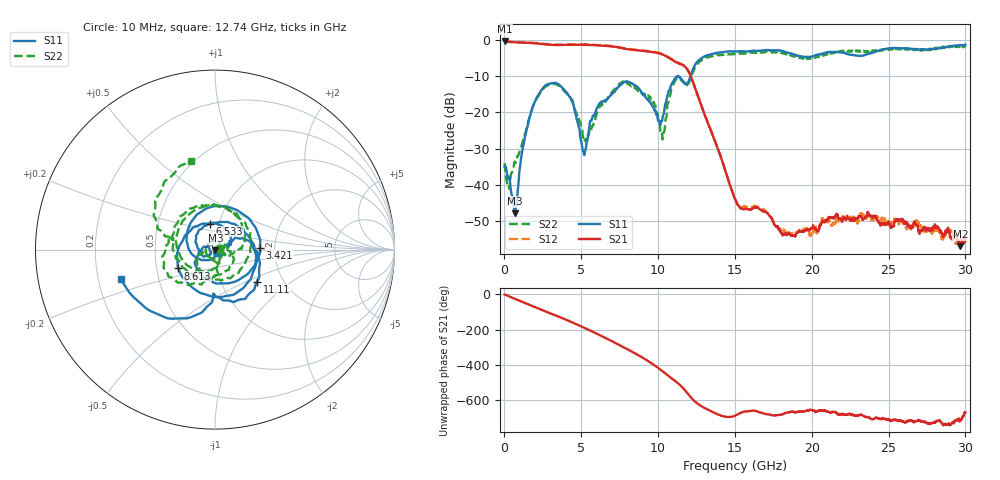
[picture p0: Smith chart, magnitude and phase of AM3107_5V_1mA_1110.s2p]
# Hz S DB R 50.0
!freq dBS11 angS11 dBS21 angS21 dBS12 angS12 dBS22 angS22
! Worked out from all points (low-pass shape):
!   1601 points, 10 MHz to 30 GHz, reference 50 ohm
!   highest |S21| = -0.16 dB at 10 MHz (marker M1); lowest = -57.1 dB at 29.68 GHz (marker M2)
!   |S21| within 3 dB of the highest: start of sweep to 9.478 GHz
!   lowest |S11| = -48.0 dB at 666 MHz (marker M3), VSWR 1.01, Z = 50.3 - j0.294 ohm
!   |S11| at or under -10 dB: start of sweep to 11.26 GHz; 11.33 GHz to 12.11 GHz (779.4 MHz wide, 6.65 % of centre)
!   |S22| runs from -41.2 to -1.5 dB; largest |S21 - S12| = 0.014
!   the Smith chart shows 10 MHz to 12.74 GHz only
!   S11 on the Smith chart (normalised r, x): 10 MHz: 1.02, -0.03; 3.421 GHz: 1.67, +0.03; 6.533 GHz: 0.91, +0.27; 8.613 GHz: 0.65, -0.14; 11.11 GHz: 1.48, -0.58; 12.74 GHz: 0.30, -0.14
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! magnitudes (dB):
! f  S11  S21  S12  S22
! 10 MHz  -35.1  -0.2  0.0  -34.1
! 253.7 MHz  -38.5  -0.4  -0.4  -40.2
! 666 MHz  -48.0  -0.6  -0.5  -33.6
! 1.809 GHz  -18.8  -0.8  -0.7  -18.8
! 3.421 GHz  -12.0  -1.3  -1.2  -12.3
! 4.377 GHz  -16.8  -1.3  -1.2  -16.6
! 5.015 GHz  -28.5  -1.3  -1.2  -24.0
! 5.352 GHz  -28.3  -1.3  -1.2  -27.9
! 6.533 GHz  -16.7  -1.5  -1.4  -16.8
! 7.695 GHz  -11.8  -2.2  -2.1  -11.4
! 8.613 GHz  -12.8  -2.8  -2.7  -13.7
! 10.02 GHz  -22.4  -3.6  -3.4  -22.2
! 10.32 GHz  -20.8  -4.0  -3.9  -26.6
! 11.11 GHz  -10.6  -5.9  -5.8  -11.1
! 11.87 GHz  -12.1  -7.9  -7.8  -12.4
! 12.74 GHz  -5.2  -17.2  -17.1  -5.8
! 15.01 GHz  -3.1  -44.0  -44.0  -3.8
! 18.14 GHz  -3.0  -54.0  -52.7  -3.6
! 20.01 GHz  -4.6  -52.2  -53.0  -5.0
! 25.01 GHz  -2.3  -50.4  -50.5  -2.6
! 29.68 GHz  -1.3  -57.1  -55.2  -1.7
! 30 GHz  -1.2  -55.4  -54.8  -1.6
